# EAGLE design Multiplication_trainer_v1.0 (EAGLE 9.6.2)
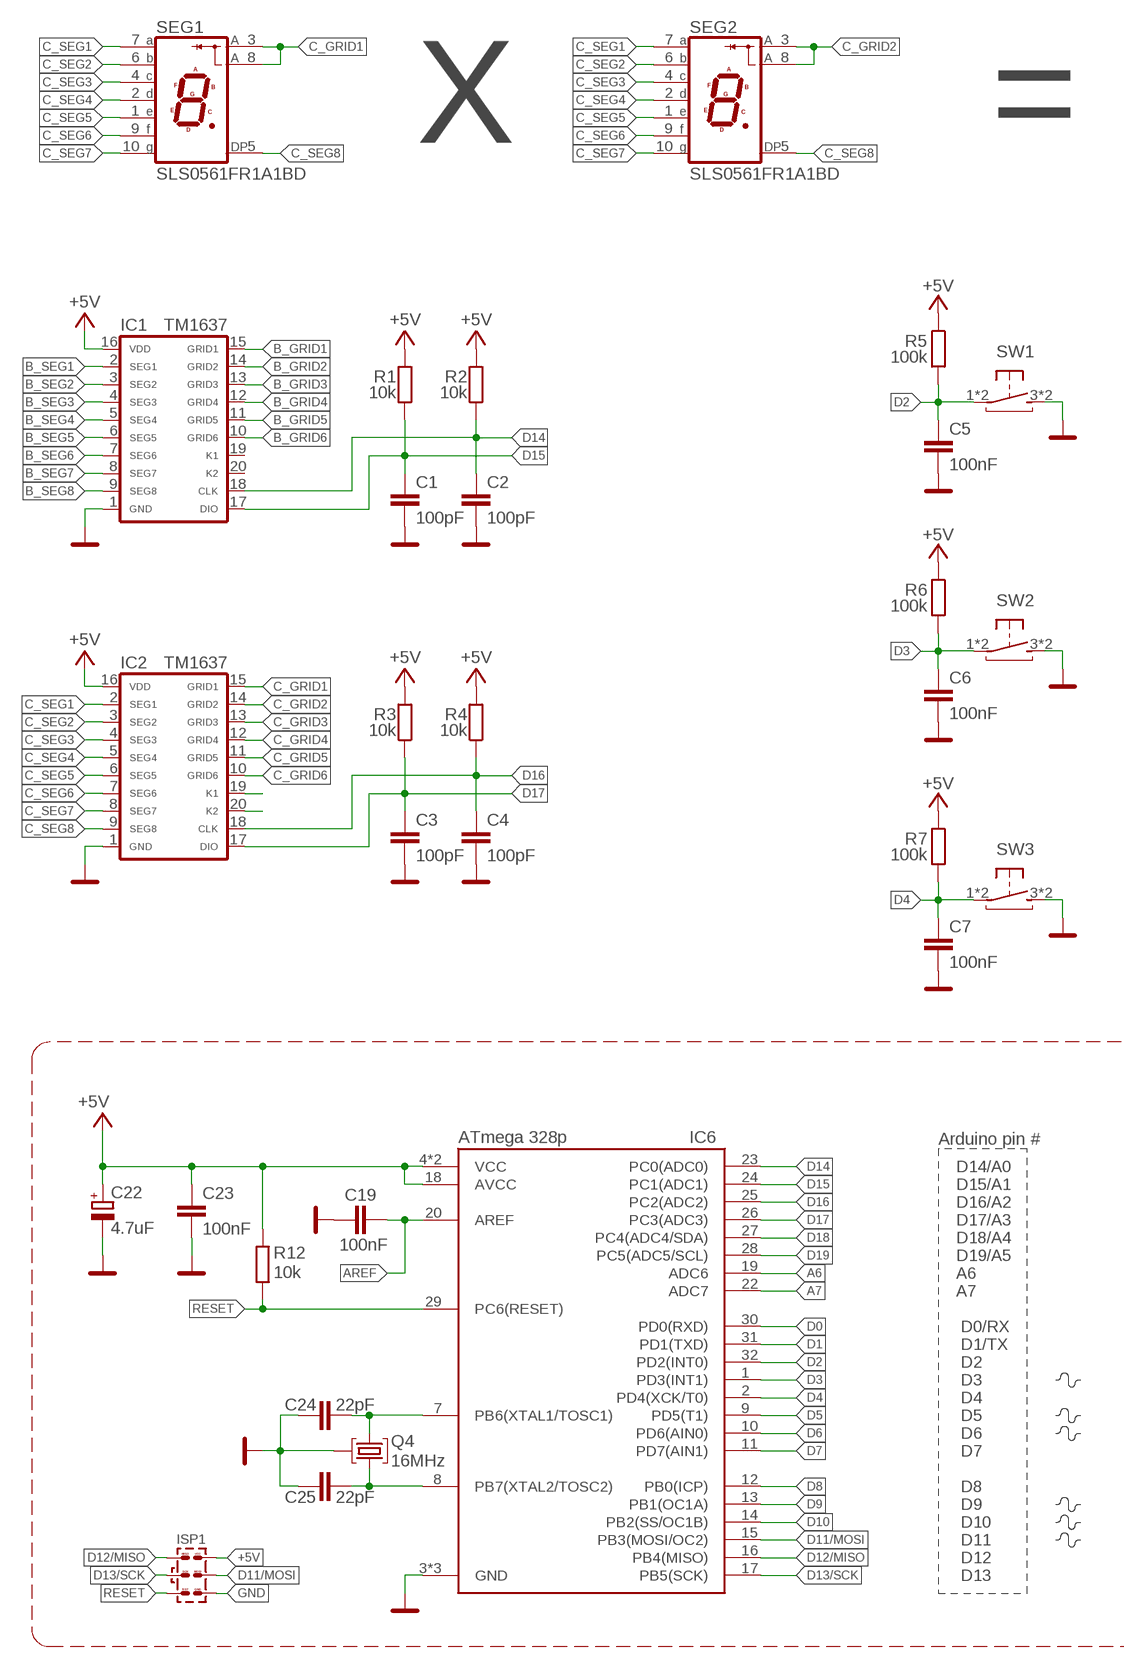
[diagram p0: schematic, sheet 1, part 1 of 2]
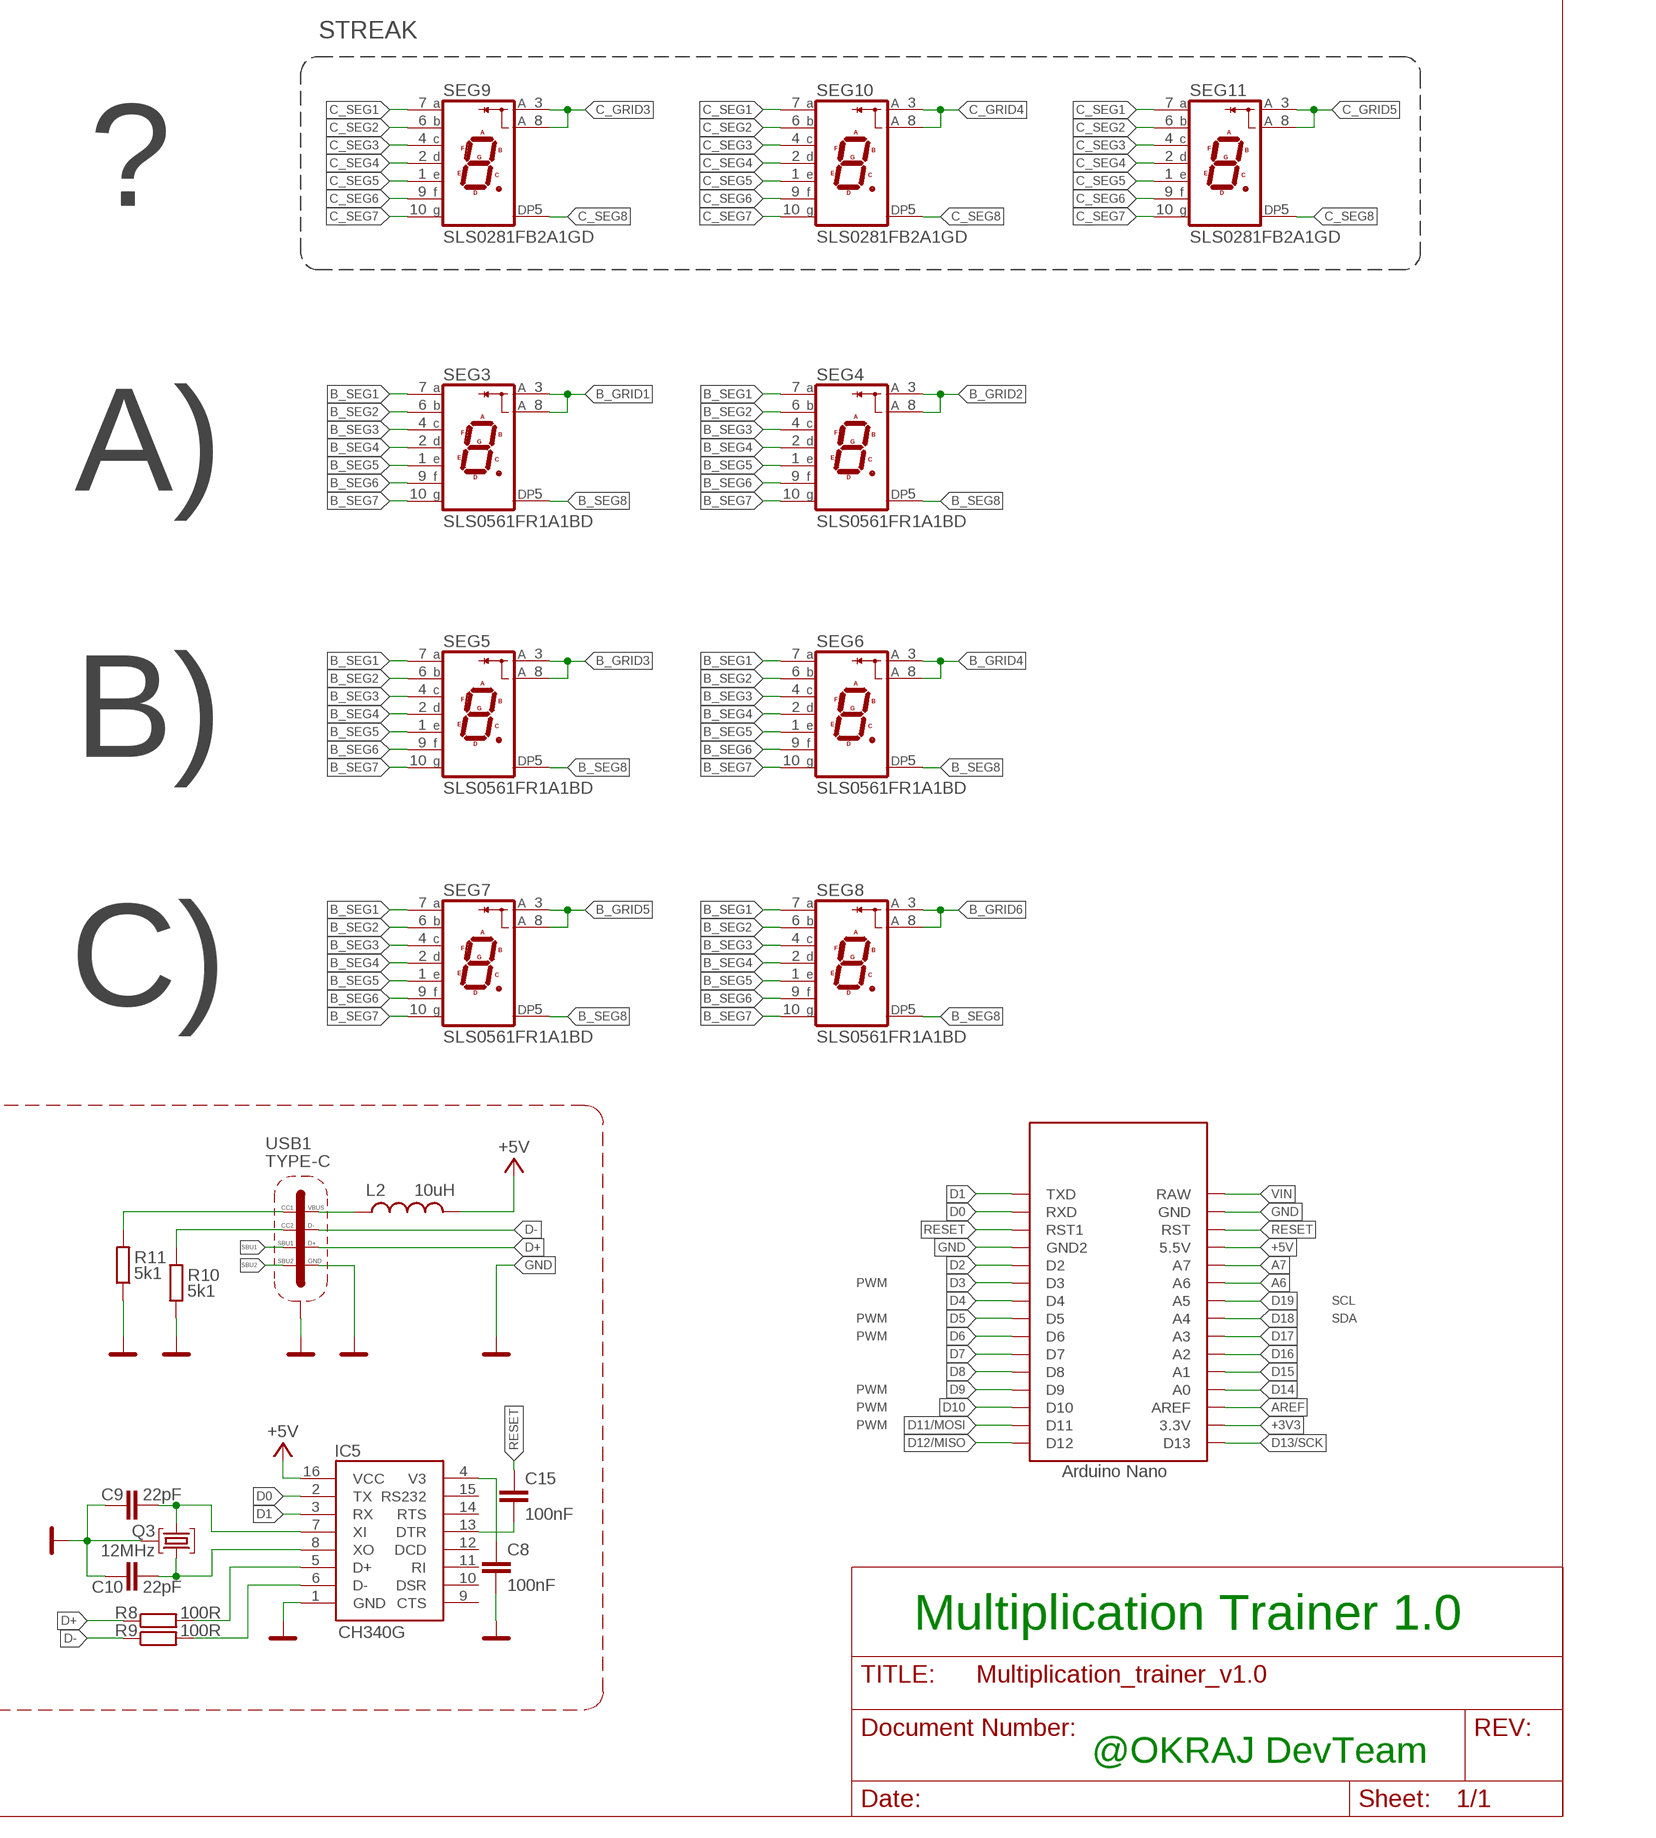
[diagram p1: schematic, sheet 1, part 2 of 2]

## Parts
C1  100pF  C-EUC0805K  [C0805K]
C2  100pF  C-EUC0805K  [C0805K]
C3  100pF  C-EUC0805K  [C0805K]
C4  100pF  C-EUC0805K  [C0805K]
C5  100nF  C-EUC0805  [C0805]
C6  100nF  C-EUC0805  [C0805]
C7  100nF  C-EUC0805  [C0805]
C8  100nF  C-EUC0603  [C0603]
C9  22pF  C-EUC0603  [C0603]
C10  22pF  C-EUC0603  [C0603]
C15  100nF  C-EUC0603  [C0603]
C19  100nF  C-EUC0603  [C0603]
C22  4.7uF  CPOL-EUSMCA  [SMC_A]
C23  100nF  C-EUC0603  [C0603]
C24  22pF  C-EUC0603  [C0603]
C25  22pF  C-EUC0603  [C0603]
IC1  TM1637  [SOP20]
IC2  TM1637  [SOP20]
IC5  CH340G  CH340GSMD  [SOIC16]
IC6  ATmega 328p  ATMEGA328PQFP32N_ROUND-PADS  [QFP80P900X900X120-32N_ROUND-PADS]
ISP1  AVR-ISP-SPI  [AVR-ISP-SPI]
L2  10uH  L-USL0805  [R0805]
Q3  12MHz  KRYSTAL  [ILCX13-FF5F18-16.0000]
Q4  16MHz  KRYSTAL  [ILCX13-FF5F18-16.0000]
R1  10k  R-EU_R0805  [R0805]
R2  10k  R-EU_R0805  [R0805]
R3  10k  R-EU_R0805  [R0805]
R4  10k  R-EU_R0805  [R0805]
R5  100k  R-EU_R0805  [R0805]
R6  100k  R-EU_R0805  [R0805]
R7  100k  R-EU_R0805  [R0805]
R8  100R  R-EU_R0603  [R0603]
R9  100R  R-EU_R0603  [R0603]
R10  5k1  R-EU_R0603  [R0603]
R11  5k1  R-EU_R0603  [R0603]
R12  10k  R-EU_R0603  [R0603]
SEG1  SLS0561FR1A1BD  [SLS0561FR1A1BD]
SEG2  SLS0561FR1A1BD  [SLS0561FR1A1BD]
SEG3  SLS0561FR1A1BD  [SLS0561FR1A1BD]
SEG4  SLS0561FR1A1BD  [SLS0561FR1A1BD]
SEG5  SLS0561FR1A1BD  [SLS0561FR1A1BD]
SEG6  SLS0561FR1A1BD  [SLS0561FR1A1BD]
SEG7  SLS0561FR1A1BD  [SLS0561FR1A1BD]
SEG8  SLS0561FR1A1BD  [SLS0561FR1A1BD]
SEG9  SLS0281FB2A1GD  [SLS0281FB2A1GD]
SEG10  SLS0281FB2A1GD  [SLS0281FB2A1GD]
SEG11  SLS0281FB2A1GD  [SLS0281FB2A1GD]
SW1  TACT-SW_BTNSMTJLC_6X6X4.5  [TACTSW_6X6X4.5_SMT]
SW2  TACT-SW_BTNSMTJLC_6X6X4.5  [TACTSW_6X6X4.5_SMT]
SW3  TACT-SW_BTNSMTJLC_6X6X4.5  [TACTSW_6X6X4.5_SMT]
U$2  NANOTHT-NOUSB  [NANO-NOUSB]
USB1  TYPE-C  TYPE-C-31-M-12TYPE-C-31_L8.94_W7.3  [TYPE-C-31_L8.94_W7.3]

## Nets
+3V3: U$2.3.3V
+5V: C22.+ C23.1 IC1.16(VDD) IC2.16(VDD) IC5.16(VCC) IC6.4(VCC) IC6.6(VCC) IC6.18(AVCC) ISP1.2 L2.2 R1.2 R2.2 R3.2 R4.2 R5.1 R6.1 R7.1 R12.1 U$2.5V(5.5V)
A6: IC6.19(ADC6) U$2.A6
A7: IC6.22(ADC7) U$2.A7
AREF: C19.1 IC6.20(AREF) U$2.AREF
B_GRID1: IC1.15(GRID1) SEG3.3(CA1) SEG3.8(CA2)
B_GRID2: IC1.14(GRID2) SEG4.3(CA1) SEG4.8(CA2)
B_GRID3: IC1.13(GRID3) SEG5.3(CA1) SEG5.8(CA2)
B_GRID4: IC1.12(GRID4) SEG6.3(CA1) SEG6.8(CA2)
B_GRID5: IC1.11(GRID5) SEG7.3(CA1) SEG7.8(CA2)
B_GRID6: IC1.10(GRID6) SEG8.3(CA1) SEG8.8(CA2)
B_SEG1: IC1.2(SEG1) SEG3.7(A) SEG4.7(A) SEG5.7(A) SEG6.7(A) SEG7.7(A) SEG8.7(A)
B_SEG2: IC1.3(SEG2) SEG3.6(B) SEG4.6(B) SEG5.6(B) SEG6.6(B) SEG7.6(B) SEG8.6(B)
B_SEG3: IC1.4(SEG3) SEG3.4(C) SEG4.4(C) SEG5.4(C) SEG6.4(C) SEG7.4(C) SEG8.4(C)
B_SEG4: IC1.5(SEG4) SEG3.2(D) SEG4.2(D) SEG5.2(D) SEG6.2(D) SEG7.2(D) SEG8.2(D)
B_SEG5: IC1.6(SEG5) SEG3.1(E) SEG4.1(E) SEG5.1(E) SEG6.1(E) SEG7.1(E) SEG8.1(E)
B_SEG6: IC1.7(SEG6) SEG3.9(F) SEG4.9(F) SEG5.9(F) SEG6.9(F) SEG7.9(F) SEG8.9(F)
B_SEG7: IC1.8(SEG7) SEG3.10(G) SEG4.10(G) SEG5.10(G) SEG6.10(G) SEG7.10(G) SEG8.10(G)
B_SEG8: IC1.9(SEG8) SEG3.5(DP) SEG4.5(DP) SEG5.5(DP) SEG6.5(DP) SEG7.5(DP) SEG8.5(DP)
C_GRID1: IC2.15(GRID1) SEG1.3(CA1) SEG1.8(CA2)
C_GRID2: IC2.14(GRID2) SEG2.3(CA1) SEG2.8(CA2)
C_GRID3: IC2.13(GRID3) SEG9.3(CA1) SEG9.8(CA2)
C_GRID4: IC2.12(GRID4) SEG10.3(CA1) SEG10.8(CA2)
C_GRID5: IC2.11(GRID5) SEG11.3(CA1) SEG11.8(CA2)
C_GRID6: IC2.10(GRID6)
C_SEG1: IC2.2(SEG1) SEG1.7(A) SEG2.7(A) SEG9.7(A) SEG10.7(A) SEG11.7(A)
C_SEG2: IC2.3(SEG2) SEG1.6(B) SEG2.6(B) SEG9.6(B) SEG10.6(B) SEG11.6(B)
C_SEG3: IC2.4(SEG3) SEG1.4(C) SEG2.4(C) SEG9.4(C) SEG10.4(C) SEG11.4(C)
C_SEG4: IC2.5(SEG4) SEG1.2(D) SEG2.2(D) SEG9.2(D) SEG10.2(D) SEG11.2(D)
C_SEG5: IC2.6(SEG5) SEG1.1(E) SEG2.1(E) SEG9.1(E) SEG10.1(E) SEG11.1(E)
C_SEG6: IC2.7(SEG6) SEG1.9(F) SEG2.9(F) SEG9.9(F) SEG10.9(F) SEG11.9(F)
C_SEG7: IC2.8(SEG7) SEG1.10(G) SEG2.10(G) SEG9.10(G) SEG10.10(G) SEG11.10(G)
C_SEG8: IC2.9(SEG8) SEG1.5(DP) SEG2.5(DP) SEG9.5(DP) SEG10.5(DP) SEG11.5(DP)
D0: IC5.2(TX) IC6.30(PD0(RXD)) U$2.RX1(RXD)
D1: IC5.3(RX) IC6.31(PD1(TXD)) U$2.TX0(TXD)
D2: C5.1 IC6.32(PD2(INT0)) R5.2 SW1.1(P) SW1.2(P) U$2.D2
D3: C6.1 IC6.1(PD3(INT1)) R6.2 SW2.1(P) SW2.2(P) U$2.D3
D4: C7.1 IC6.2(PD4(XCK/T0)) R7.2 SW3.1(P) SW3.2(P) U$2.D4
D5: IC6.9(PD5(T1)) U$2.D5
D6: IC6.10(PD6(AIN0)) U$2.D6
D7: IC6.11(PD7(AIN1)) U$2.D7
D8: IC6.12(PB0(ICP)) U$2.D8
D9: IC6.13(PB1(OC1A)) U$2.D9
D10: IC6.14(PB2(SS/OC1B)) U$2.D10
D11/MOSI: IC6.15(PB3(MOSI/OC2)) ISP1.4 U$2.D11
D12/MISO: IC6.16(PB4(MISO)) ISP1.1 U$2.D12
D13/SCK: IC6.17(PB5(SCK)) ISP1.3 U$2.D13
D14: C2.1 IC1.18(CLK) IC6.23(PC0(ADC0)) R2.1 U$2.A0
D15: C1.1 IC1.17(DIO) IC6.24(PC1(ADC1)) R1.1 U$2.A1
D16: C4.1 IC2.18(CLK) IC6.25(PC2(ADC2)) R4.1 U$2.A2
D17: C3.1 IC2.17(DIO) IC6.26(PC3(ADC3)) R3.1 U$2.A3
D18: IC6.27(PC4(ADC4/SDA)) U$2.A4
D19: IC6.28(PC5(ADC5/SCL)) U$2.A5
D+: R8.1 USB1.A6(D+) USB1.B6(D+)
D-: R9.1 USB1.A7(D-) USB1.B7(D-)
GND: C1.2 C2.2 C3.2 C4.2 C5.2 C6.2 C7.2 C8.2 C9.2 C10.2 C19.2 C22.- C23.2 C24.2 C25.2 IC1.1(GND) IC2.1(GND) IC5.1(GND) IC6.3(GND) IC6.5(GND) IC6.21(GND) ISP1.6 Q3.P$2(GND) Q3.P$4(GND) Q4.P$2(GND) Q4.P$4(GND) R10.1 R11.1 SW1.3(S) SW1.4(S) SW2.3(S) SW2.4(S) SW3.3(S) SW3.4(S) U$2.GND U$2.GND1(GND2) USB1.A1/B12(GND) USB1.B1/A12(GND) USB1.SHIELD1(SHIELD) USB1.SHIELD2(SHIELD) USB1.SHIELD3(SHIELD) USB1.SHIELD4(SHIELD) USB1.SHIELD5(SHIELD) USB1.SHIELD6(SHIELD) USB1.SHIELD7(SHIELD) USB1.SHIELD8(SHIELD)
N$1: C8.1 IC5.4(V3)
N$2: C9.1 IC5.7(XI) Q3.P$1
N$3: C10.1 IC5.8(XO) Q3.P$3
N$4: C15.2 IC5.13(DTR)
N$5: IC5.5(D+) R8.2
N$6: IC2.19(K1)
N$7: IC2.20(K2)
N$8: IC5.6(D-) R9.2
N$9: L2.1 USB1.A4/B9(VBUS) USB1.B4/A9(VBUS)
N$10: R10.2 USB1.B5(CC2)
N$11: R11.2 USB1.A5(CC1)
N$12: C24.1 IC6.7(PB6(XTAL1/TOSC1)) Q4.P$1
N$13: C25.1 IC6.8(PB7(XTAL2/TOSC2)) Q4.P$3
RESET: C15.1 IC6.29(PC6(RESET)) ISP1.5 R12.2 U$2.RST U$2.RST1
SBU1: USB1.A8(SBU1)
SBU2: USB1.B8(SBU2)
VIN: U$2.RAW
Unconnected: IC1.19(K1) IC1.20(K2) IC5.9(CTS) IC5.10(DSR) IC5.11(RI) IC5.12(DCD) IC5.14(RTS) IC5.15(RS232)

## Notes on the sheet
- STREAK
- X | = | ?
- A)
- B)
- C)
- Arduino pin #
- D14/A0
- D15/A1
- D16/A2
- D17/A3 | PWM
- D18/A4 | SCL
- D19/A5 | PWM | SDA
- A6 | PWM
- A7
- D0/RX | PWM
- D1/TX | PWM
- D2 | PWM
- D3
- D4
- D5
- D6
- D7
- D8
- D9
- D10
- D11
- D12
- Multiplication Trainer 1.0
- D13
- @OKRAJ DevTeam

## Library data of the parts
C1-C4 = rcl:C-EU: CAPACITOR, European symbol; LCSC_PART: C1790; SPICEPREFIX: C
C5-C7 = rcl:C-EU: CAPACITOR, European symbol
C8 C15 C19 C23 = rcl:C-EU: CAPACITOR, European symbol; LCSC_PART: C49678; SPICEPREFIX: C
C9 C10 C24 C25 = rcl:C-EU: CAPACITOR, European symbol; LCSC_PART: C1804; SPICEPREFIX: C
C22 = rcl:CPOL-EU: POLARIZED CAPACITOR, European symbol; LCSC_PART: C111040; ROT: 180; SPICEPREFIX: C
IC1 IC2 = #my:TM1637; LCSC_PART: C20001; ROT: 270
IC5 = ch340g:CH340G; LCSC_PART: C14267
IC6 = ATMEGA328P-ANR:ATMEGA328P: 8-bit Microcontrollers - MCU AVR 32K FLSH 2K SRAM 1KB EE-20 MHZ 105C Source: Datasheet; LCSC_PART: C14877; ROT: 270
ISP1 = #Ondra2:AVR-ISP-SPI
L2 = rcl:L-US: INDUCTOR, American symbol; LCSC_PART: C281113
Q3 = #Marek:KRYSTAL: Monolithic Crystal Filters Source: www.vanlong.com; LCSC_PART: C9002
Q4 = #Marek:KRYSTAL: Monolithic Crystal Filters Source: www.vanlong.com; LCSC_PART: C13738
R1-R4 R8 R9 R12 = rcl:R-EU_: RESISTOR, European symbol; SPICEPREFIX: R
R5-R7 = resistor:R-EU_: RESISTOR, European symbol
R10 R11 = rcl:R-EU_: RESISTOR, European symbol; LCSC_PART: C27834; SPICEPREFIX: R
SEG1-SEG8 = #my:SLS0561FR1A1BD; LCSC_PART: C226002
SEG9-SEG11 = #my:SLS0281FB2A1GD; LCSC_PART: C225995
SW1-SW3 = #Ondra2:TACT-SW_BTN; LCSC_PART: C127509
U$2 = Arduino-clone:NANO: Arduino Nano
USB1 = #Marek:TYPE-C-31-M-12; LCSC_PART: C165948; ROT: 180

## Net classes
0 default: width 0.127 mm, drill 0.2 mm, clearance 0.127 mm

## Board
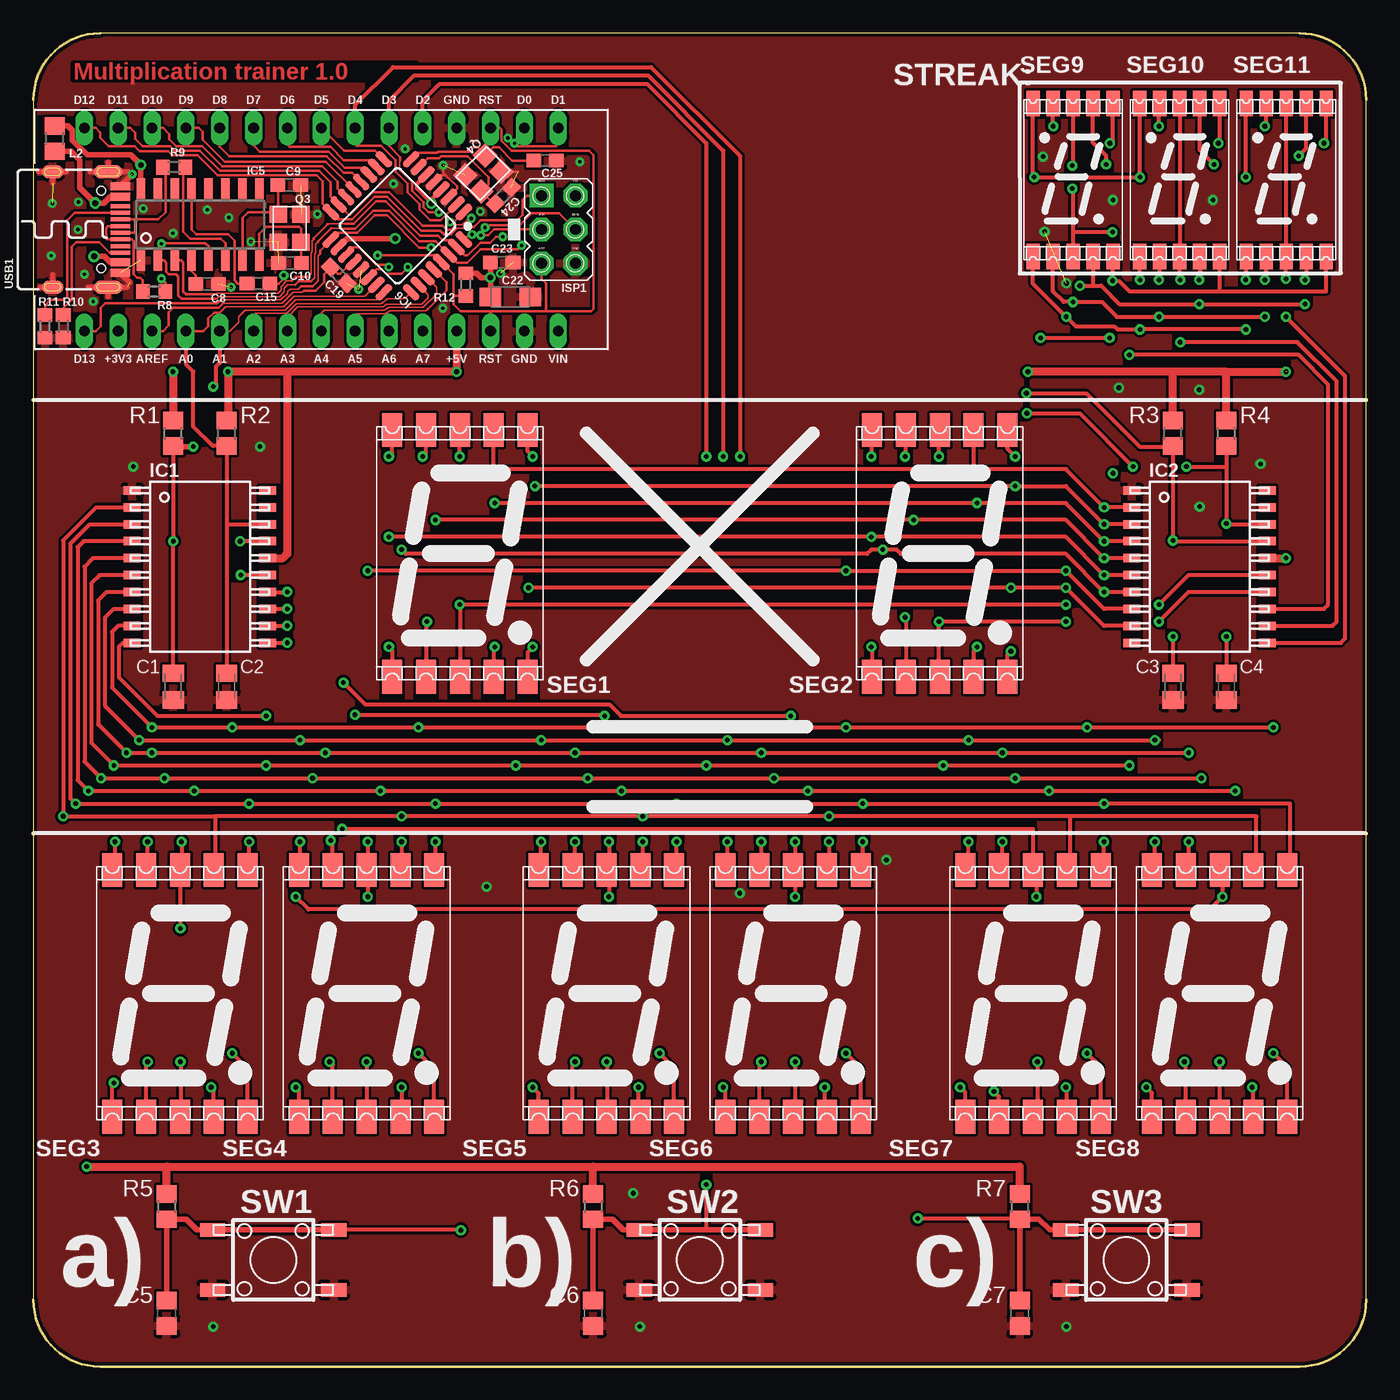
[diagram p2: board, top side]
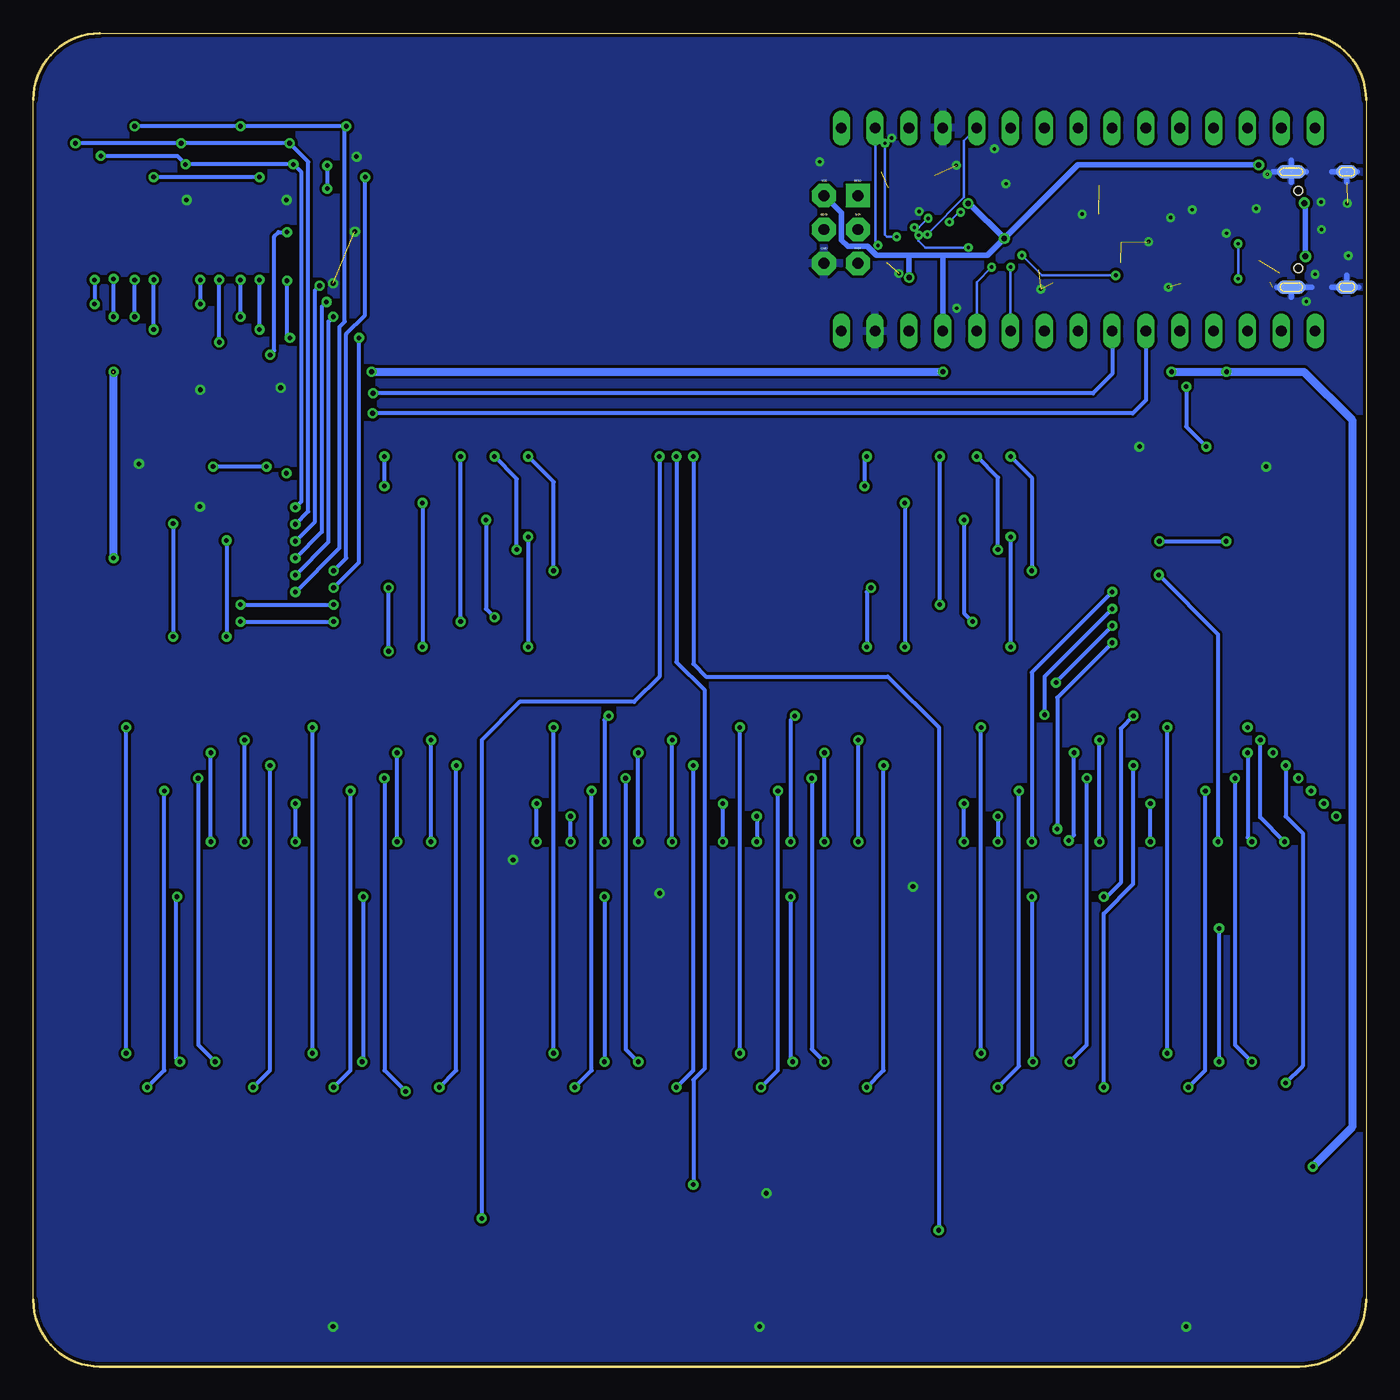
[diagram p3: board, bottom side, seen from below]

Size 100 x 100 mm. Coordinates in mm from the lower left corner, seen from the top.
Outline: 100,5 100,95 arc90 95,100 5,100 arc90 0,95 0,5 arc90 5,0 95,0 arc90 100,5
Copper layers (1*16): Top 0.035mm / dielectric 1.5mm / Bottom 0.035mm
Design rules "default": minimum track width 10mil, minimum drill 24mil, track to track 8mil, track to pad 8mil, pad to pad 8mil, via to via 8mil, smd to smd 8mil, copper to edge 10mil, drill to drill 8mil, minimum pad ring 10mil, minimum via ring 8mil, stop-mask expansion 4mil, vias tented up to drill 0.7mm, thermal gap 10mil

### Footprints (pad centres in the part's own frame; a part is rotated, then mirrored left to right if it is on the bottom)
C0805K = smd 1.3 x 1.6: 1 -1,0; 2 1,0
C0805 = smd 1.3 x 1.5: 1 -0.95,0; 2 0.95,0
C0603 = smd 1.1 x 1: 1 -0.85,0; 2 0.85,0
SMC_A = smd 1.6 x 1.4: + -1.5,0; - 1.5,0
SOP20 = smd 1.27 x 0.635: 1 -5.08,5.715; 2 -5.08,4.445; 3 -5.08,3.175; 4 -5.08,1.905; 5 -5.08,0.635; 6 -5.08,-0.635; 7 -5.08,-1.905; 8 -5.08,-3.175; 9 -5.08,-4.445; 10 -5.08,-5.715; 11 5.08,-5.715; 12 5.08,-4.445; 13 5.08,-3.175; 14 5.08,-1.905; 15 5.08,-0.635; 16 5.08,0.635; 17 5.08,1.905; 18 5.08,3.175; 19 5.08,4.445; 20 5.08,5.715
SOIC16 = smd 0.635 x 1.524: 1 -4.445,-2.695; 2 -3.175,-2.695; 3 -1.905,-2.695; 4 -0.635,-2.695; 5 0.635,-2.695; 6 1.905,-2.695; 7 3.175,-2.695; 8 4.445,-2.695; 9 4.445,2.695; 10 3.175,2.695; 11 1.905,2.695; 12 0.635,2.695; 13 -0.635,2.695; 14 -1.905,2.695; 15 -3.175,2.695; 16 -4.445,2.695
QFP80P900X900X120-32N_ROUND-PADS = smd 1.499 x 0.584: 1 -4.25,2.8; 2 -4.25,2; 3 -4.25,1.2; 4 -4.25,0.4; 5 -4.25,-0.4; 6 -4.25,-1.2; 7 -4.25,-2; 8 -4.25,-2.8; 17 4.25,-2.8; 18 4.25,-2; 19 4.25,-1.2; 20 4.25,-0.4; 21 4.25,0.4; 22 4.25,1.2; 23 4.25,2; 24 4.25,2.8 | smd 0.584 x 1.499: 9 -2.8,-4.25; 10 -2,-4.25; 11 -1.2,-4.25; 12 -0.4,-4.25; 13 0.4,-4.25; 14 1.2,-4.25; 15 2,-4.25; 16 2.8,-4.25; 25 2.8,4.25; 26 2,4.25; 27 1.2,4.25; 28 0.4,4.25; 29 -0.4,4.25; 30 -1.2,4.25; 31 -2,4.25; 32 -2.8,4.25
AVR-ISP-SPI = drill 0.813 pad 1.778 square: 1 -1.27,2.54 | drill 0.813 pad 1.778 octagon: 2 1.27,2.54; 3 -1.27,0; 4 1.27,0; 5 -1.27,-2.54; 6 1.27,-2.54
R0805 = smd 1.3 x 1.5: 1 -0.95,0; 2 0.95,0
ILCX13-FF5F18-16.0000 = smd 1.3 x 1.3: P$1 -1.05,-0.85; P$2 1.05,-0.85; P$3 1.05,0.85; P$4 -1.05,0.85
R0603 = smd 1 x 1.1: 1 -0.85,0; 2 0.85,0
SLS0561FR1A1BD = smd 1.5 x 2.54: 1 -5.08,-9.25; 2 -2.54,-9.25; 3 0,-9.25; 4 2.54,-9.25; 5 5.08,-9.25; 6 5.08,9.25; 7 2.54,9.25; 8 0,9.25; 9 -2.54,9.25; 10 -5.08,9.25
SLS0281FB2A1GD = smd 1 x 1.905: 1 -3,-5.75; 2 -1.5,-5.75; 3 0,-5.75; 4 1.5,-5.75; 5 3,-5.75; 6 3,5.75; 7 1.5,5.75; 8 0,5.75; 9 -1.5,5.75; 10 -3,5.75
TACTSW_6X6X4.5_SMT = smd 1.9 x 1: 1 -4.55,2.25; 2 4.55,2.25; 3 -4.55,-2.25; 4 4.55,-2.25
NANO-NOUSB = drill 0.8 long: 3.3V -7.62,15.24; 5V -7.62,-10.16; A0 -7.62,10.16; A1 -7.62,7.62; A2 -7.62,5.08; A3 -7.62,2.54; A4 -7.62,0; A5 -7.62,-2.54; A6 -7.62,-5.08; A7 -7.62,-7.62; AREF -7.62,12.7; D2 7.62,-7.62; D3 7.62,-5.08; D4 7.62,-2.54; D5 7.62,0; D6 7.62,2.54; D7 7.62,5.08; D8 7.62,7.62; D9 7.62,10.16; D10 7.62,12.7; D11 7.62,15.24; D12 7.62,17.78; D13 -7.62,17.78; GND -7.62,-15.24; GND1 7.62,-10.16; RAW -7.62,-17.78; RST -7.62,-12.7; RST1 7.62,-12.7; RX1 7.62,-15.24; TX0 7.62,-17.78
TYPE-C-31_L8.94_W7.3 = smd 0.6 x 1.45: A1/B12 -3.25,3.885; A4/B9 -2.45,3.885; B1/A12 3.25,3.885; B4/A9 2.45,3.885 | smd 0.3 x 1.45: A5 -1.25,3.885; A6 -0.25,3.885; A7 0.25,3.885; A8 1.25,3.885; B5 1.75,3.885; B6 0.75,3.885; B7 -0.75,3.885; B8 -1.75,3.885 | smd 1 x 2.1: SHIELD1 -4.32,2.97; SHIELD2 4.32,2.97 | smd 1 x 1.6: SHIELD3 -4.32,-1.21; SHIELD4 4.32,-1.21 | smd 1 x 2.1 bottom: SHIELD5 -4.316,2.97; SHIELD8 4.316,2.97 | smd 1 x 1.6 bottom: SHIELD6 -4.316,-1.21; SHIELD7 4.316,-1.21 | hole 0.65: -2.89,2.44; 2.89,2.44

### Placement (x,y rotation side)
C1  10.5,51 270 top
C2  14.5,51 270 top
C3  85.5,51 270 top
C4  89.5,51 270 top
C5  10,4 270 top
C6  42,4 270 top
C7  74,4 270 top
C8  13.04,81.2 0 top
C9  19.19,88.62 0 top
C10  19.25,82.78 180 top
C15  16.89,81.24 180 top
C19  22.91,81.85 315 top
C22  35.79,80.23 0 top
C23  35.14,82.82 0 top
C24  35.26,87.83 45 top
C25  38.39,90.46 0 top
IC1  12.5,60 0 top
IC2  87.5,60 0 top
IC5  12.51,85.66 0 top
IC6  27.31,85.56 225 top
ISP1  39.4,85.29 0 top
L2  1.59,92.11 90 top
Q3  19.22,85.38 270 top
Q4  33.75,89.49 45 top
R1  10.5,70 90 top
R2  14.5,70 90 top
R3  85.5,70 90 top
R4  89.5,70 90 top
R5  10,12 270 top
R6  42,12 270 top
R7  74,12 270 top
R8  9.06,80.62 0 top
R9  10.56,89.96 0 top
R10  2.24,78.02 90 top
R11  0.87,78.02 90 top
R12  32.44,81.15 270 top
SEG1  32,61 0 top
SEG2  68,61 0 top
SEG3  11,28 0 top
SEG4  25,28 0 top
SEG5  43,28 0 top
SEG6  57,28 0 top
SEG7  75,28 0 top
SEG8  89,28 0 top
SEG9  78,89 0 top
SEG10  86,89 0 top
SEG11  94,89 0 top
SW1  18,8 0 top
SW2  50,8 0 top
SW3  82,8 0 top
U$2  21.6,85.29 90 top
USB1  2.64,85.29 270 top

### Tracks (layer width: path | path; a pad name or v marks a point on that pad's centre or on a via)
+5V  (via drill 0.35, 0.35 pad 0.55, 0.4)  (1 unrouted)
  Top 0.305: IC6.4 29.84,87.52 | 29.85,87.52 29.84,87.52 | 29.84,87.52 29.62,87.52 28.78,88.36 28.78,88.73 IC6.6
  Top 0.406: L2.2 2.59,93.06 2.93,92.72 2.93,91.98 4.02,90.88 7.3,90.88 v8.06,90.13 IC5.16 | IC6.18 23.52,84.6 27.13,84.6 v27.15,84.61 | v29.85,87.24 29.85,87.52 | C22.+ v34.29,81.67 | v34.29,81.67 v34.29,81.68 | C23.1 v34.29,81.67 | v34.29,81.67 | R12.1 33.25,82 33.58,81.67 v34.29,81.67
  Top 0.61: U$2.5V 31.75,77.66 v31.75,74.61 19.05,74.61 | R3.2 85.5,74.61 | v10.48,74.61 10.48,70.97 R1.2 | R2.2 14.61,71.06 v14.61,74.61 19.05,74.61 | R5.1 10,15 | R6.1 42,15 | R7.1 74,15 42,15 | v4,15 10,15 | 10,15 42,15 | 89.53,74.61 85.5,74.61 | 89.53,74.61 94.03,74.61 | IC1.16 18.73,60.63 19.05,60.96 19.05,74.61 | IC2.16 v93.97,60.63 v93.98,60.64 | R4.2 89.5,74.58 89.53,74.61 | 85.5,74.61 v74.61,74.61
  Bottom 0.406: v27.15,84.61 29.77,87.24 v29.85,87.24 | v27.15,84.61 28.42,83.34 31.75,83.34 | v34.29,81.68 34.29,83.26 34.21,83.34 | 31.75,83.34 34.21,83.34 | 34.21,83.34 36.74,83.34 37.42,84.02 38.89,84.02 39.37,84.5 39.37,86.53 ISP1.2 | v27.15,84.61 21.63,90.13 v8.06,90.13 | U$2.5V 31.76,83.33 31.75,83.34
  Bottom 0.61: v4,15 1.05,17.95 1.05,71 4.66,74.61 v10.48,74.61 v14.61,74.61 | v93.98,60.64 v93.98,74.61 | v74.61,74.61 v31.75,74.61
A6  (via drill 0.25)
  Top 0.203: IC6.19 24.02,83.96 24.39,83.96 25.72,82.63 26.51,82.63 v26.67,82.47
  Bottom 0.203: U$2.A6 v26.68,82.47 v26.67,82.47
A7  (via drill 0.25)
  Top 0.203: IC6.22 25.75,82.3 26.13,82.3 26.44,81.98 27.61,81.98 v28.09,82.46 v28.1,82.46
  Bottom 0.203: U$2.A7 29.22,81.34 v28.1,82.46
AREF
  Top 0.127: 13.89,79.42 14.22,79.75 18.67,79.75 19.49,80.57 20.16,80.57 20.3,80.71
  Top 0.203: U$2.AREF 9.72,77.67 10.16,78.1 10.16,79.09 10.49,79.42 13.89,79.42 | 20.3,80.71 21.16,80.71 21.8,81.34 21.8,81.94 C19.1 22.81,81.95 23.02,81.95 23.91,82.84 IC6.20
B_GRID1  (via drill 0.35 pad 0.55)
  Top 0.305: IC1.15 v15.56,59.37 | v11.11,39.37 11.11,37.36 SEG3.8 11,32.89 v11.03,32.86 | v11.03,22.86 11.03,18.78 SEG3.3
  Bottom 0.305: v15.56,59.37 11.11,54.93 v11.11,39.37 | v11.03,32.86 v11.03,22.86
B_GRID2  (via drill 0.35 pad 0.55)
  Top 0.305: IC1.14 v19.04,58.09 v19.05,58.1 | v25.08,39.37 25.08,37.33 SEG4.8 25.08,37.17 v25.08,35.25 v25.08,35.24 | v25,22.86 SEG4.3
  Bottom 0.305: v19.05,58.1 25.08,52.07 v25.08,39.37 | v25.08,35.24 25.08,22.94 v25,22.86
B_GRID3  (via drill 0.35 pad 0.55)
  Top 0.305: IC1.13 v19.05,56.83 | v24.13,48.9 42.77,48.9 v42.86,48.81 | v43.18,39.37 43.18,37.43 SEG5.8 43.18,37.07 v43.18,35.24 | v43.02,22.86 43.02,18.77 SEG5.3
  Bottom 0.305: v19.05,56.83 24.13,51.75 v24.13,48.9 | v42.86,48.81 43.18,48.49 v43.18,39.37 | v43.18,35.24 43.18,23.02 v43.02,22.86
B_GRID4  (via drill 0.35 pad 0.55)
  Top 0.305: IC1.12 v19.04,55.55 v19.05,55.56 | v56.83,48.81 44.08,48.81 43.22,49.67 24.89,49.67 v23.27,51.3 | v57.15,39.37 57.15,37.4 SEG6.8 57.15,37.1 v57.15,35.24 | v57.15,22.86 57.15,18.9 SEG6.3
  Bottom 0.305: v19.05,55.56 23.27,51.35 v23.27,51.3 | v56.83,48.81 57.15,48.49 v57.15,39.37 | v57.15,35.24 v57.15,22.86
B_GRID5  (via drill 0.35 pad 0.55)
  Top 0.305: IC1.11 v19.04,54.28 v19.05,54.29 | v23.18,40.32 75,40.32 SEG7.8 75.25,37 v75.25,35.24 | v75.33,22.86 75.33,19.08 SEG7.3
  Bottom 0.305: v19.05,54.29 23.18,50.16 v23.18,40.32 | v75.25,35.24 75.25,22.94 v75.33,22.86
B_GRID6  (via drill 0.35 pad 0.55)
  Top 0.305: IC1.10 6.72,54.28 6.41,53.98 6.41,51.69 9.3,48.81 v17.46,48.81 | v19.68,35.24 20.64,34.29 88.27,34.29 v89.22,35.24 89.22,37.03 SEG8.8 | SEG8.3 v89,22.86
  Bottom 0.305: v17.46,48.81 18.41,47.85 18.41,36.27 19.45,35.24 v19.68,35.24 | v89.22,35.24 89.32,35.14 89.32,23.18 v89,22.86
B_SEG1  (via drill 0.35 pad 0.55)
  Top 0.305: IC1.2 7.41,64.45 4.72,64.45 2.23,61.96 v2.23,41.27 13.65,41.27 | 77.79,41.27 91.76,41.27 91.76,37.47 SEG8.7 | 77.79,41.27 v59.69,41.27 v45.72,41.27 v27.62,41.27 13.65,41.27 | 13.65,41.27 13.65,37.36 SEG3.7 | v27.62,39.37 27.62,37.33 SEG4.7 | v45.72,39.37 45.72,37.43 SEG5.7 | v59.69,39.37 59.69,37.4 SEG6.7 | SEG7.7 77.79,37.5 77.79,41.27
  Bottom 0.305: v27.62,41.27 v27.62,39.37 | v45.72,41.27 v45.72,39.37 | v59.69,39.37 v59.69,41.27
B_SEG2  (via drill 0.35 pad 0.55)
  Top 0.305: IC1.3 4.24,63.17 2.78,61.72 2.78,42.63 v3.17,42.23 v16.19,42.23 v30.16,42.23 v48.26,42.23 v62.23,42.23 v80.33,42.23 94.3,42.23 94.3,37.47 SEG8.6 | SEG3.6 16.19,37.36 v16.19,39.37 | SEG4.6 30.16,37.33 v30.16,39.37 | SEG5.6 48.26,37.43 v48.26,39.37 | SEG6.6 62.23,37.4 v62.23,39.37 | SEG7.6 80.33,37.5 v80.33,39.37
  Bottom 0.305: v16.19,39.37 v16.19,42.23 | v30.16,39.37 v30.16,42.23 | v48.26,39.37 v48.26,42.23 | v62.23,39.37 v62.23,42.23 | v80.33,39.37 v80.33,42.23
B_SEG3  (via drill 0.35 pad 0.55)
  Top 0.305: IC1.4 3.76,61.91 3.32,61.47 3.32,43.98 v4.13,43.18 v12.06,43.18 v26.04,43.18 v44.13,43.18 v58.1,43.18 v76.2,43.18 v90.17,43.18 | SEG3.4 13.54,20.75 v13.34,20.95 | v27.62,20.95 27.62,18.83 SEG4.4 | SEG5.4 45.4,18.89 v45.4,20.95 | SEG6.4 59.37,18.92 v59.37,20.95 | SEG7.4 77.54,20.89 v77.47,20.95 | SEG8.4 91.54,20.86 v91.44,20.95
  Bottom 0.305: v13.34,20.95 12.06,22.23 v12.06,43.18 | v27.62,20.95 26.04,22.54 v26.04,43.18 | v45.4,20.95 44.13,22.23 v44.13,43.18 | v59.37,20.95 58.1,22.23 v58.1,43.18 | v77.47,20.95 76.2,22.23 v76.2,43.18 | v91.44,20.95 90.17,22.23 v90.17,43.18
B_SEG4  (via drill 0.35 pad 0.55)
  Top 0.305: IC1.5 4.46,60.63 3.83,60.01 3.83,45.38 v5.08,44.13 v9.84,44.13 v20.95,44.13 v41.59,44.13 v55.56,44.13 v73.66,44.13 v87.63,44.13 | SEG3.2 8.46,22.75 v8.57,22.86 | SEG4.2 22.46,22.62 v22.23,22.86 | SEG5.2 40.46,22.68 v40.64,22.86 | SEG6.2 54.46,22.71 v54.61,22.86 | SEG7.2 72.46,20.25 v72.07,20.64 | SEG8.2 86.46,22.76 v86.36,22.86
  Bottom 0.305: v9.84,44.13 9.84,24.13 v8.57,22.86 | v22.23,22.86 20.95,24.13 v20.95,44.13 | v40.64,22.86 41.59,23.81 v41.59,44.13 | v55.56,44.13 55.56,23.81 v54.61,22.86 | v72.07,20.64 73.66,22.23 v73.66,44.13 | v87.63,44.13 87.63,24.13 v86.36,22.86
B_SEG5  (via drill 0.35 pad 0.55)
  Top 0.305: IC1.6 4.97,59.37 4.34,58.74 4.34,46.78 v6.03,45.09 v17.46,45.09 v36.2,45.09 v50.48,45.09 v68.26,45.09 v82.23,45.09 | v6.03,21.27 5.92,21.16 SEG3.1 | SEG4.1 19.92,20.72 v19.68,20.95 | SEG5.1 37.92,20.5 v37.47,20.95 | SEG6.1 51.92,20.79 v51.75,20.95 | SEG7.1 69.92,20.57 v69.53,20.95 | SEG8.1 83.92,20.54 v83.5,20.95
  Bottom 0.305: v6.03,21.27 4.76,22.54 4.76,40.01 6.03,41.27 v6.03,45.09 | v19.68,20.95 19.68,33.97 17.46,36.2 v17.46,45.09 | v37.47,20.95 36.2,22.23 v36.2,45.09 | v51.75,20.95 50.48,22.23 v50.48,45.09 | v69.53,20.95 68.26,22.23 v68.26,45.09 | v83.5,20.95 82.23,22.23 v82.23,45.09
B_SEG6  (via drill 0.35 pad 0.55)
  Top 0.305: IC1.7 5.47,58.09 4.85,57.47 4.85,48.18 v6.99,46.04 v8.89,46.04 v21.91,46.04 v40.64,46.04 v54.61,46.04 v72.71,46.04 v86.68,46.04 | SEG3.9 8.57,37.36 v8.57,39.37 | SEG4.9 22.46,39.32 v22.32,39.46 | SEG5.9 40.64,37.43 v40.64,39.37 | SEG6.9 54.61,37.4 v54.61,39.37 | SEG7.9 72.71,37.5 v72.71,39.37 | SEG8.9 86.68,37.47 v86.68,39.37
  Bottom 0.305: v8.89,46.04 8.89,39.69 v8.57,39.37 | v22.32,39.46 21.91,39.87 v21.91,46.04 | v40.64,39.37 v40.64,46.04 | v54.61,39.37 v54.61,46.04 | v72.71,39.37 v72.71,46.04 | v86.68,39.37 v86.68,46.04
B_SEG7  (via drill 0.35 pad 0.55)
  Top 0.305: IC1.8 6.03,56.83 5.4,56.2 5.4,49.53 v7.94,46.99 v20,46.99 v38.1,46.99 v52.07,46.99 v70.17,46.99 v84.14,46.99 84.45,46.99 | SEG3.10 6.12,37.45 v6.12,39.37 | SEG4.10 20,37.33 v20,39.37 | SEG5.10 38.1,37.43 v38.1,39.37 | SEG6.10 52.07,37.4 v52.07,39.37 | SEG7.10 70.17,37.5 v70.17,39.37 | SEG8.10 84.14,37.47 v84.14,39.37
  Bottom 0.305: v6.12,39.37 7.94,41.19 v7.94,46.99 | v20,39.37 v20,46.99 | v38.1,39.37 v38.1,46.99 | v52.07,39.37 v52.07,46.99 | v70.17,39.37 v70.17,46.99 | v84.14,39.37 v84.14,46.99
B_SEG8  (via drill 0.35 pad 0.55)
  Top 0.305: IC1.9 6.36,55.55 5.91,55.1 5.91,50.93 v8.89,47.94 v14.92,47.94 v28.89,47.94 v46.99,47.94 v60.96,47.94 v79.06,47.94 v93.03,47.94 | SEG3.5 16.08,22.34 v14.92,23.5 | SEG5.5 48.08,22.41 v46.99,23.5 | SEG4.5 30.08,22.31 v28.89,23.5 | SEG6.5 62.08,22.38 v60.96,23.5 | SEG7.5 80.08,22.47 v79.06,23.5 | SEG8.5 94.08,22.44 v93.03,23.5
  Bottom 0.305: v14.92,23.5 v14.92,47.94 | v46.99,23.5 v46.99,47.94 | v28.89,23.5 v28.89,47.94 | v60.96,23.5 v60.96,47.94 | v79.06,23.5 v79.06,47.94 | v93.03,23.5 v93.03,47.94
C_GRID1  (via drill 0.35)
  Top 0.305: IC2.15 86.67,59.37 v84.45,57.15 | v31.99,68.26 31.99,70.24 SEG1.8 | v77.47,57.15 v31.99,57.15 32,57.14 SEG1.3
  Bottom 0.305: v84.45,57.15 v77.47,57.15 | v31.99,57.15 v31.99,68.26
C_GRID2  (via drill 0.35)
  Top 0.305: IC2.14 86.67,58.09 v84.45,55.88 | v77.47,55.88 v67.94,55.88 67.94,51.8 SEG2.3 | v67.94,68.26 67.94,70.19 SEG2.8
  Bottom 0.305: v84.45,55.88 v77.47,55.88 | v67.94,55.88 v67.94,68.26
C_GRID3  (via drill 0.35)
  Top 0.305: IC2.13 96.83,56.83 97.16,57.15 97.16,73.66 94.93,75.88 v82.23,75.88 | SEG9.8 78,90.14 v77.95,90.08 | v77.95,88.35 78,88.3 78,85.09 | 78,85.09 SEG9.3 | v80.96,85.09 78,85.09
  Bottom 0.305: v77.95,90.08 v77.95,88.35 | v82.23,75.88 81.92,76.2 81.92,84.77 81.6,85.09 v80.96,85.09
C_GRID4  (via drill 0.35)
  Top 0.305: IC2.12 97.47,55.55 97.79,55.88 97.79,73.89 94.85,76.83 v86.04,76.83 | SEG10.8 86,83.5 SEG10.3 86,81.55 v86.04,81.51
  Bottom 0.305: v86.04,76.83 v86.04,81.51
C_GRID5  (via drill 0.35)
  Top 0.305: IC2.11 98.1,54.28 98.42,54.61 98.42,74.3 v93.98,78.74 | v93.98,81.58 93.98,83.23 SEG11.3 SEG11.8
  Bottom 0.305: v93.98,78.74 v93.98,81.58
C_SEG1  (via drill 0.35)
  Top 0.305: IC2.2 v80.33,64.44 77.47,67.31 70.54,67.31 | 70.54,67.31 34.61,67.31 34.54,67.38 SEG1.7 | SEG2.7 70.54,67.31 | v80.49,90.17 80.49,90.81 79.5,91.79 SEG9.7 | v94.93,90.81 95.5,91.37 SEG11.7 | v88.58,90.17 87.5,91.25 SEG10.7
  Bottom 0.305: v80.33,64.44 79.88,64.9 79.88,89.57 v80.49,90.17 v88.58,90.17 89.22,90.81 v94.93,90.81
C_SEG2  (via drill 0.35)
  Top 0.305: IC2.3 v80.33,63.17 77.47,66.04 v73.66,66.04 v37.62,66.04 | 73.03,70.19 SEG2.6 73.08,68.84 v73.66,68.26 | v37.47,68.26 37.08,68.65 SEG1.6 | v80.77,91.76 81,91.99 SEG9.6 | v88.9,91.76 89,91.86 SEG10.6 | v96.84,91.76 97,91.92 SEG11.6
  Bottom 0.305: v73.66,66.04 v73.66,68.26 | v37.62,66.04 37.62,68.1 v37.47,68.26 | v80.33,63.17 79.38,64.14 79.38,90.37 v80.77,91.76 v88.9,91.76 v96.84,91.76
C_SEG3  (via drill 0.35)
  Top 0.305: IC2.4 v80.33,61.91 77.47,64.77 v70.8,64.77 v34.61,64.77 | v70.8,53.98 70.54,53.71 SEG2.4 | v34.61,53.98 34.54,53.91 SEG1.4 | 78.69,81.07 v78.51,81.07 79.53,81.07 | 79.53,81.07 80.11,81.07 81.49,79.69 v87.47,79.69 v95.41,79.69 | 79.53,81.07 79.5,81.1 SEG9.4 | SEG10.4 87.5,81.54 v87.47,81.51 | SEG11.4 95.5,81.6 v95.41,81.51
  Bottom 0.305: v70.8,64.77 v70.8,53.98 | v34.61,64.77 v34.61,53.98 | v80.33,61.91 78.87,63.37 78.87,80.71 v78.51,81.07 | v87.47,81.51 v87.47,79.69 | v95.41,81.51 v95.41,79.69
C_SEG4  (via drill 0.35)
  Top 0.305: IC2.5 v80.33,60.63 77.47,63.5 v66.04,63.5 v30.16,63.5 | v65.41,56.2 65.46,56.14 SEG2.2 | v29.53,55.88 29.46,55.81 SEG1.2 | SEG9.2 76.5,80.66 77.31,79.85 v78,79.85 80.17,79.85 81.28,78.74 v84.45,78.74 v92.39,78.74 | v92.39,81.51 92.5,81.62 SEG11.2 | v84.45,81.51 84.5,81.55 SEG10.2
  Bottom 0.305: v66.04,63.5 66.04,56.83 v65.41,56.2 | v30.16,63.5 30.16,56.52 v29.53,55.88 | v80.33,60.63 78.36,62.61 78.36,79.5 v78,79.85 | v92.39,78.74 v92.39,81.51 | v84.45,78.74 v84.45,81.51
C_SEG5  (via drill 0.35)
  Top 0.305: IC2.6 v80.33,59.37 77.47,62.23 v62.87,62.23 v26.67,62.23 | v62.87,53.98 62.92,53.92 SEG2.1 | v26.67,53.98 26.92,53.73 SEG1.1 | SEG9.1 75,81.21 77.47,78.74 v77.5,78.74 78.22,78.02 81.1,78.02 81.33,77.79 v83.03,77.79 v90.96,77.79 | v83.03,81.51 83,81.53 SEG10.1 | SEG11.1 90.96,83.21 v90.96,81.52
  Bottom 0.305: v62.87,62.23 v62.87,53.98 | v26.67,62.23 v26.67,53.98 | v80.33,59.37 77.85,61.85 77.85,78.38 v77.5,78.74 | v83.03,77.79 v83.03,81.51 | v90.96,77.79 v90.96,81.51 v90.96,81.52
C_SEG6  (via drill 0.35)
  Top 0.305: IC2.7 v80.33,58.09 77.47,60.96 65.09,60.96 64.77,61.28 v63.73,61.28 62.87,61.28 62.55,60.96 27.94,60.96 v27.62,61.28 | v65.41,68.26 65.46,68.32 SEG2.9 | v29.21,68.26 29.46,68.51 SEG1.9 | v76.52,93.03 76.5,93.05 SEG9.9 | v84.45,93.03 84.45,94.7 SEG10.9 | v92.39,93.03 92.5,93.14 SEG11.9
  Bottom 0.305: v63.73,61.28 63.73,66.59 v65.41,68.26 | v27.62,61.28 27.62,66.67 v29.21,68.26 | v80.33,58.09 77.03,61.4 77.03,77.99 76.63,78.38 76.63,92.91 v76.52,93.03 v84.45,93.03 v92.39,93.03
C_SEG7  (via drill 0.35)
  Top 0.305: IC2.8 80.33,56.83 v77.47,59.69 v60.96,59.69 v25.08,59.69 | v26.67,68.26 26.92,68.51 SEG1.10 | v62.87,68.26 62.92,68.32 SEG2.10 | SEG9.10 75,89.31 v75.09,89.22 v83.03,89.22 83.03,94.72 SEG10.10 | v90.96,89.22 90.96,94.71 SEG11.10
  Bottom 0.305: v26.67,68.26 25.08,66.67 v25.08,59.69 | v60.96,59.69 60.96,66.36 v62.87,68.26 | v77.47,59.69 76.52,60.64 76.52,77.46 75.11,78.87 75.11,89.2 v75.09,89.22 | v83.03,89.22 v90.96,89.22
C_SEG8  (via drill 0.35)
  Top 0.305: IC2.9 80.33,55.55 v77.47,58.42 v73.34,58.42 v37.15,58.42 | v37.47,53.98 37.08,53.59 SEG1.5 | SEG2.5 73.08,53.4 v73.34,53.66 | SEG9.5 81,81.48 v80.96,81.44 81.44,81.44 82.23,80.64 88.9,80.64 | 88.9,80.64 97,80.64 SEG11.5 | 88.9,80.64 89,80.75 SEG10.5 | v75.56,77.15 v80.75,77.15
  Bottom 0.305: v37.15,58.42 37.47,58.1 v37.47,53.98 | v73.34,53.66 v73.34,58.42 | v80.75,77.15 80.96,77.37 v80.96,81.44 | v77.47,58.42 75.56,60.33 v75.56,77.15
D0  (via drill 0.25)
  Top 0.127: 22.35,85.4 23.2,85.4 23.24,85.36 | 13.65,80.08 13.73,80.08 13.91,80.26 18.46,80.26 18.82,80.62 18.82,80.88 19.08,81.14 19.63,81.14 | 20.82,81.39 21.09,81.66 21.09,83.42 21.17,83.5 21.17,84.17 21.37,84.37
  Top 0.203: 13.65,80.08 11.11,80.08 10.87,80.32 10.87,81.76 10.72,81.92 10.16,81.92 9.97,82.11 9.97,82.8 9.81,82.96 IC5.2 | v36.63,84.1 36.35,83.81 33.55,83.81 32.53,82.79 31.79,82.79 IC6.30 30.16,84.42 28.93,84.42 26.67,86.68 25.47,86.68 24.15,85.36 23.24,85.36 | 22.35,85.4 21.37,84.41 21.37,84.37 | 19.63,81.14 19.89,81.39 20.82,81.39
  Bottom 0.203: v36.63,84.1 36.83,84.3 36.83,92.9 U$2.RX1
D1  (via drill 0.25)
  Top 0.127: 22.03,85.68 22.07,85.72 23.36,85.72 23.37,85.72 | 13.57,80.41 13.65,80.41 13.75,80.51 18.36,80.51 18.57,80.73 18.57,80.98 19.02,81.43 19.38,81.43 | 20.62,81.74 20.84,81.96 20.84,83.53 20.91,83.61 20.91,84.43 21.03,84.54
  Top 0.203: 21.03,84.54 21.03,84.62 22.09,85.68 22.03,85.68 | 23.37,85.72 24.03,85.72 25.72,87.41 26.41,87.41 29.01,84.81 30.38,84.81 30.72,84.47 31.24,84.47 IC6.31 32.37,83.34 32.57,83.34 33.53,84.3 34.27,84.3 34.71,84.74 v35.23,84.74 | v36.1,91.76 36.34,91.52 39.22,91.52 39.38,91.68 U$2.TX0 | 20.62,81.74 19.69,81.74 19.38,81.43 | IC5.3 11.08,82.96 11.24,82.8 11.24,80.62 11.44,80.41 13.57,80.41
  Bottom 0.203: v35.23,84.74 35.95,84.74 36.1,84.89 v36.1,91.76
D2  (via drill 0.25, 0.35)
  Top 0.203: IC6.32 32.66,84.9 32.91,84.9 v32.92,84.91
  Top 0.305: U$2.D2 29.22,94.94 30.48,96.2 46.04,96.2 50.48,91.76 v50.48,68.26 | v32.07,10.23 32.05,10.25 SW1.2
  Top 0.406: SW1.2 SW1.1 12.25,10.25 11.45,11.05 R5.2 C5.1
  Bottom 0.203: v32.92,84.91 32.78,85.04 32.78,85.1 30.17,87.7 30.17,91.95 U$2.D2
  Bottom 0.305: v32.07,10.23 32.07,47.94 35.88,51.75 49.53,51.75 50.48,52.7 v50.48,68.26
D3  (via drill 0.25, 0.35)
  Top 0.127: 27.55,89.7 27.46,89.79 27.46,90.45 27.51,90.5
  Top 0.203: IC6.1 31.64,85.93 31.34,85.93 v31.26,85.85 | v30.41,86.58 29.66,86.58 29.29,86.94 29.29,87.31 28.4,88.21 28.4,88.86 27.55,89.7 | 27.51,90.5 27.51,90.72 26.68,91.56 U$2.D3
  Top 0.305: U$2.D3 26.68,94.94 28.57,96.84 46.12,96.84 51.75,91.21 v51.75,68.26 | v50.48,13.65 50.48,10.25
  Top 0.406: C6.1 R6.2 43.45,11.05 44.25,10.25 SW2.1 50.48,10.25 SW2.2
  Bottom 0.203: v31.26,85.85 30.54,86.58 v30.41,86.58
  Bottom 0.305: v51.75,68.26 51.75,52.84 49.62,50.71 49.62,22.37 50.48,21.51 v50.48,13.65
D4  (via drill 0.35)
  Top 0.203: U$2.D4 24.14,91.67 24.25,91.56 26.07,91.56 27.16,90.48 27.16,89.63 28.07,88.72 28.07,88.07 28.96,87.18 28.96,86.81 28.97,86.8 28.97,86.76 29.77,85.96 30.54,85.96 IC6.2
  Top 0.305: U$2.D4 24.14,94.62 26.99,97.47 46.35,97.47 53.02,90.81 v53.02,68.26 | v66.36,11.11 73.94,11.11 R7.2
  Top 0.406: SW3.2 SW3.1 76.25,10.25 75.45,11.05 R7.2 C7.1
  Bottom 0.305: v53.02,68.26 53.02,51.75 54.93,49.85 63.5,49.85 66.36,46.99 v66.36,11.11
D5
  Top 0.203: IC6.9 25.64,91.2 23.3,91.2 U$2.D5
D6
  Top 0.203: IC6.10 25.21,90.5 23.29,90.5 22.31,91.48 19.22,91.48 19.06,91.64 U$2.D6
D7
  Top 0.203: IC6.11 25.11,89.42 24.6,89.93 23.34,89.93 22.16,91.12 16.99,91.12 16.52,91.59 U$2.D7
D8
  Top 0.203: U$2.D8 13.98,91.5 14.68,90.79 22.02,90.79 23.28,89.53 23.92,89.53 IC6.12
D9
  Top 0.203: U$2.D9 12.42,92.91 12.7,92.62 12.7,92.02 14.33,90.38 21.93,90.38 IC6.13
D10
  Top 0.203: IC6.14 22.84,88.34 22.84,88.86 21.67,90.04 14.17,90.04 12.67,91.54 10.71,91.54 10.2,92.06 10.2,92.43 9.72,92.91 U$2.D10
D11/MOSI  (via drill 0.25)
  Top 0.127: 32.31,85.77 32.18,85.64 31.68,85.64 31.32,85.28 31.29,85.28
  Top 0.203: U$2.D11 7.25,92.91 7.63,92.53 7.63,92.08 8.18,91.53 10.26,91.53 10.58,91.21 12.48,91.21 14,89.69 21.45,89.69 22.3,88.84 22.3,87.75 IC6.15 23.66,86.39 23.76,86.39 25.43,88.06 26.68,88.06 29.18,85.57 30.72,85.57 31.01,85.28 31.29,85.28 | v32.86,86.12 32.66,86.12 32.31,85.77 | v33.89,85.44 34.07,85.62 36.48,85.62 37.39,86.52 39.44,86.52 ISP1.4
  Bottom 0.203: v32.86,86.12 33.55,85.44 v33.89,85.44
D12/MISO
  Top 0.127: 31.35,84.93 31.8,85.38 32.38,85.38
  Top 0.203: U$2.D12 4.67,92.91 5.02,92.56 5.02,92.16 5.64,91.53 7.6,91.53 7.97,91.16 10.12,91.16 10.42,90.86 12.32,90.86 13.82,89.35 21.24,89.35 21.69,88.9 21.69,87.23 IC6.16 22.87,86.05 23.9,86.05 25.58,87.73 26.55,87.73 28.43,85.86 29.08,85.2 30.53,85.2 30.8,84.93 31.35,84.93 | ISP1.1 37.03,87.83 36.71,87.51 36.71,86.4 36.28,85.97 33.53,85.97 33.03,85.46 32.46,85.46 32.38,85.38
D13/SCK  (via drill 0.25)
  Top 0.127: 13.73,79.75 13.81,79.75 14.06,80 18.57,80 19.08,80.52 19.08,80.64 19.26,80.82 19.87,80.82 20.08,81.04 | 20.95,81.04 21.35,81.44 21.35,83.32 21.5,83.47
  Top 0.203: U$2.D13 4.67,77.67 5.05,78.05 5.05,79.43 5.37,79.75 13.73,79.75 | 21.5,83.47 21.5,83.71 IC6.17 22.82,85.03 24.29,85.03 25.61,86.35 26.53,86.35 28.95,83.93 v29.84,83.93 | v33.58,84.85 34.13,84.85 34.57,85.29 ISP1.3 | 20.08,81.04 20.95,81.04
  Bottom 0.203: v29.84,83.93 33.05,83.93 33.58,84.45 v33.58,84.85
D14
  Top 0.127: 13.97,79.06 14.41,79.5 18.78,79.5 19.57,80.29 24.86,80.29 IC6.23
  Top 0.203: U$2.A0 12.75,77.67 13.11,78.02 13.11,78.61 13.55,79.06 13.97,79.06
  Top 0.305: 14.5,63.25 R2.1 13.45,69.05 12,70.5 12,74.63 11.44,75.19 U$2.A0 | IC1.18 14.57,63.17 14.5,63.25 | 14.5,63.25 C2.1
D15  (via drill 0.35, 0.35 pad 0.55)
  Top 0.127: U$2.A1 14.72,77.67 15.4,78.34 15.4,78.74 15.9,79.24 18.88,79.24 19.66,80.02 25.73,80.02 IC6.24
  Top 0.305: C1.1 v10.5,61.91 10.5,69 R1.1 | IC1.17 v15.52,61.91 | U$2.A1 13.98,75.28 13.69,74.99 13.69,73.69
  Top 0.406: 13.69,73.69 v13.5,73.5 | v12,69 10.5,69
  Bottom 0.305: v15.52,61.91 v10.5,61.91 | v13.5,73.5 13.5,70.5 v12,69
D16  (via drill 0.35)
  Top 0.127: U$2.A2 16.52,78.84 16.67,78.99 18.99,78.99 19.73,79.73 26.02,79.73 arc45 26.24,79.82 26.42,80 arc-45 26.64,80.09 27.85,80.09 IC6.25
  Top 0.305: R4.1 89.5,67.5 | 89.5,67.5 v89.5,63.23 89.56,63.17 IC2.18 | v89.5,54.75 C4.1 | v74.54,71.5 78.5,71.5 v82.5,67.5 | v86.5,67.5 89.5,67.5
  Bottom 0.305: v89.5,63.23 v89.5,54.75 | U$2.A2 16.52,72.48 17.5,71.5 v74.54,71.5 | v82.5,67.5 v86.5,67.5
D17  (via drill 0.35)
  Top 0.127: U$2.A3 19.06,78.7 19.83,79.47 26.12,79.47 arc45 26.35,79.57 26.38,79.6 arc-45 26.61,79.69 29.13,79.69 29.61,80.17 29.61,80.41 28.91,81.11 IC6.26
  Top 0.305: R3.1 85.5,69 | 85.5,69 v85.5,61.96 85.56,61.91 IC2.17 | v85.5,54.75 C3.1 | v74.5,73 79,73 83,69 85.5,69
  Bottom 0.305: v85.5,61.96 v85.5,54.75 | U$2.A3 19.05,77.65 19.05,74.45 20.5,73 v74.5,73
D18
  Top 0.127: U$2.A4 21.6,78.99 21.83,79.22 26.23,79.22 arc45 26.45,79.31 26.49,79.35 arc-45 26.71,79.44 29.24,79.44 30.24,80.44 30.24,80.94 IC6.27
D19
  Top 0.127: U$2.A5 24.14,78.86 24.25,78.97 26.33,78.97 arc45 26.56,79.06 26.59,79.09 arc-45 26.82,79.18 29.47,79.18 29.58,79.29
  Top 0.203: IC6.28 31,81.31 31,80.71 29.58,79.29
D+
  Top 0.203: USB1.A6 5.59,85.54 5.45,85.4 5.45,84.61 5.53,84.54 USB1.B6 7.38,84.54 7.51,84.4 7.51,81.94 7.78,81.68 8.02,81.68 8.21,81.48 R8.1
D-
  Top 0.203: USB1.A7 7.56,85.04 7.64,85.12 7.64,85.9 7.58,85.96 7.5,86.04 | 7.5,86.04 USB1.B7 | R9.1 9.92,89.75 9.92,86.6 9.36,86.04 7.5,86.04
GND  (via drill 0.25, 0.35)  (16 unrouted)
  Top 0.203: IC6.3 31.77,88.33 31.77,88.52 30.91,89.37 | 30.91,89.37 30.56,89.37 IC6.5 | 30.91,89.37 30.75,89.54 v30.75,90.1 | Q4.P$2 36.37,89.64
  Top 0.406: 1.43,81.9 USB1.SHIELD4 0.51,80.97 | USB1.SHIELD2 7.02,80.97 | USB1.SHIELD2 5.61,80.25 | USB1.SHIELD2 4.13,80.97 | USB1.SHIELD3 2.48,89.61 | USB1.SHIELD3 | USB1.SHIELD3 1.43,88.78 | USB1.SHIELD3 0.4,89.61 | USB1.B1/A12 7.22,81.34 | USB1.A1/B12 7.35,89.36 | 7.35,89.36 7.38,89.39 | USB1.SHIELD1 5.61,90.31 | USB1.SHIELD1 7.11,89.61 7.35,89.36 | USB1.SHIELD1 4.25,89.61
  Bottom 0.406: USB1.SHIELD6 1.43,88.82 | USB1.SHIELD6 0.66,89.6 | USB1.SHIELD6 2.58,89.6 | USB1.SHIELD5 4.48,89.6 | USB1.SHIELD5 7,89.6 | USB1.SHIELD5 5.62,88.82 | USB1.SHIELD5 | 5.61,90.47 USB1.SHIELD5 | USB1.SHIELD2 5.61,80.21 | USB1.SHIELD2 6.71,80.97 | USB1.SHIELD2 4.08,80.97 | USB1.SHIELD4 1.43,81.86 | USB1.SHIELD4 2.57,80.97 | USB1.SHIELD4 0.56,80.97
  other vias: 14.84,80.96 16.31,84.38 21.31,86.44 24.41,80.8 33.54,86.64 27.89,91.33 10.48,85.01 4.48,79.89 3.37,87.35 3.33,85.29 41,90.37 30.72,79.38 35.6,92.15 35.04,81.99 27.02,88.71 7.41,89.43 8.24,86.85 13.05,86.77 14.67,86.17 3.84,81.93 1.42,87.25 1.34,83.32 17,69 34,36 45,13 64,38 53,35.5 92.08,67.71 87.47,73.26 81.44,73.42 87.5,64.5 81,87.5 88.5,87.5 75.75,90.75 77.5,81.25 75.88,85.12 13.5,3 45.5,3 77.5,3 7.5,67.5
  pour Top: -0.5,100.5 -0.5,-0.5 100.5,-0.5 100.5,100.5
  pour Bottom: 100.5,100.5 100.5,-0.5 -0.5,-0.5 -0.5,100.5
N$1
  Top 0.203: C8.1 12.19,81.84 11.87,82.15 IC5.4
N$2
  Top 0.203: C9.1 18.34,86.58 18.23,86.58 | 18.23,86.58 Q3.P$1 | IC5.7 15.68,86.17 16.1,86.58 18.23,86.58
N$3
  Top 0.203: C10.1 20.1,84.31 Q3.P$3 20.07,85.34 19.92,85.49 17.46,85.49 16.95,84.98 IC5.8
N$4
  Top 0.203: C15.2 15.32,81.24 15.08,81.47 15.08,84.45 14.61,84.93 12.22,84.93 11.87,85.28 IC5.13
N$5  (via drill 0.25)
  Top 0.203: IC5.5 13.14,84.01 12.88,84.27 9.66,84.27 v9.6,84.22 | R8.2 9.91,81.29 v9.6,81.6
  Bottom 0.203: v9.6,81.6 v9.6,84.22
N$8
  Top 0.203: IC5.6 14.41,84.25 14.06,84.6 11.75,84.6 11.25,85.1 11.25,89.79 R9.2
N$9  (via drill 0.45)
  Top 0.406: USB1.A4/B9 5.75,87.74 5.28,87.27 v4.63,87.27 3.49,88.42 3.49,90.49 2.82,91.16 L2.1 | USB1.B4/A9 5.75,82.84 5.32,83.27 v4.55,83.27
  Bottom 0.406: v4.55,83.27 4.55,87.19 v4.63,87.27
N$10
  Top 0.203: USB1.B5 5.74,83.54 4.95,84.33 3.21,84.33 2.87,83.99 2.87,80.02 2.24,79.39 R10.2
N$11
  Top 0.203: USB1.A5 3.11,86.54 2.54,85.97 2.54,80.25 2.3,80.01 1.27,80.01 0.87,79.61 R11.2
N$12
  Top 0.203: C24.1 34.56,87.19 Q4.P$1 34.14,88.69 34.14,89.21 32.56,90.79 30.58,90.79 30.43,90.64 29.56,90.64 IC6.7
N$13
  Top 0.203: IC6.8 28.83,91.04 30.29,91.04 30.37,91.13 32.71,91.13 33.02,91.44 33.37,91.44 33.84,90.97 33.84,90.89 Q4.P$3 34.49,91.44 34.92,91.44 35.91,90.46 C25.1
N$18  (via drill 0.35)
  other vias: 81,67
RESET  (via drill 0.25, 0.3)
  Top 0.203: v25.82,83.35 v25.83,83.34 30.1,83.34 IC6.29 31.51,81.93 31.51,80.29 | C15.1 18.41,81.24 18.79,81.61 v18.79,81.85 | 31.51,80.29 31.51,79.69 32.05,79.16 34.29,79.16 | R12.2 31.52,80.3 31.51,80.29 | 38.46,79.16 34.29,79.16 | ISP1.5 38.13,81.57 38.46,81.24 38.46,79.16 | U$2.RST 34.3,79.15 34.29,79.16 | U$2.RST1 34.97,92.91 35.12,92.76 35.12,91.95 35.88,91.19 41.69,91.19 42.03,90.84 42.03,79.33 41.85,79.16 38.46,79.16
  Bottom 0.203: v18.79,81.85 24.32,81.85 v25.82,83.35

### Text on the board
Top: Multiplication trainer 1.0
tPlace: STREAK: | D12 | D11 | D10 | D9 | D8 | D7 | D6 | D5 | D4 | D3 | D2 | GND | RST | D0 | D1 | D13 | +3V3 | AREF | A0 | A1 | A2 | A3 | A4 | A5 | A6 | A7 | +5V | RST | GND | VIN | a) | b) | c)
